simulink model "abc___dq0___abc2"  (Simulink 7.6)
settings: Solver=ode23tb  StartTime=0.0  StopTime=10/f  FixedStep=Ts  RelTol=1e-3
InitFcn:
  | clear all
  | f=60;
  | %Ts=2e-5;
  | clc
  | close all
  | a=exp(j*2*pi/3);
undefined symbols (not defined in the file or in its folder): j
libraries: powerlib_extras x5

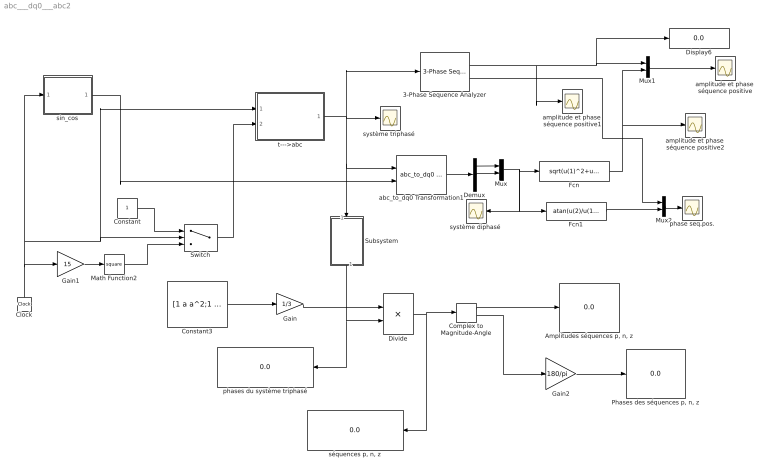
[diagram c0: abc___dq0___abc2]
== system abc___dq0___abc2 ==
  3-Phase Sequence Analyzer : powerlib_extras/Measurements/3-Phase Sequence Analyzer  DialogController=POWERSYS.PowerSysDialog  SystemSampleTime=-1  f1=60  n=1  seq=Positive
  "Amplitudes séquences p, n, z" : Display
  Clock : Clock
  Complex to Magnitude-Angle : ComplexToMagnitudeAngle  SampleTime=0
  Constant : Constant
  Constant3 : Constant  Value=[1 a a^2;1 a^2 a; 1 1 1]
  Demux : Demux  Outputs=3
  Display6 : Display
  Divide : Product  Inputs=**  Multiplication=Matrix(*)
  Fcn : Fcn  Expr=sqrt(u(1)^2+u(2)^2)
  Fcn1 : Fcn  Expr=atan(u(2)/u(1))
  Gain : Gain  Gain=1/3
  Gain1 : Gain  Gain=15
  Gain2 : Gain  Gain=180/pi
  Math Function2 : Math  Operator=square
  Mux : Mux  Inputs=2
  Mux1 : Mux  Inputs=2
  Mux2 : Mux  Inputs=2
  "Phases des séquences p, n, z" : Display
  Subsystem : Subsystem
  Switch : Switch  Threshold=3/f
  abc_to_dq0 Transformation1 : powerlib_extras/Measurements/abc_to_dq0 Transformation  DialogController=POWERSYS.PowerSysDialog  SystemSampleTime=-1
  amplitude et phase  séquence positive : Scope
  amplitude et phase  séquence positive1 : Scope
  amplitude et phase  séquence positive2 : Scope
  phase seq.pos. : Scope
  phases du système triphasé : Display
  sin_cos : Subsystem
  "système diphasé " : Scope
  "système triphasé " : Scope
  "séquences p, n, z" : Display
  t--->abc : Subsystem
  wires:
  t--->abc/1(abc) -> "système triphasé "/1, 3-Phase Sequence Analyzer/1, abc_to_dq0 Transformation1/1, Subsystem/1(syst)
  sin_cos/1(sin_cos) -> abc_to_dq0 Transformation1/2
  Gain1/1 -> Math Function2/1
  Constant/1 -> Switch/1
  Math Function2/1 -> Switch/3
  Switch/1 -> t--->abc/2(a)
  Clock/1 -> Gain1/1, sin_cos/1(t), Switch/2, t--->abc/1(t)
  Fcn1/1 -> Mux2/2
  Mux1/1 -> amplitude et phase  séquence positive/1
  3-Phase Sequence Analyzer/1 -> amplitude et phase  séquence positive1/1, Mux1/1, Display6/1
  Mux2/1 -> phase seq.pos./1
  3-Phase Sequence Analyzer/2 -> Mux2/1
  Fcn/1 -> Mux1/2, amplitude et phase  séquence positive2/1
  abc_to_dq0 Transformation1/1 -> Demux/1
  Demux/1 -> Mux/1
  Mux/1 -> Fcn/1, Fcn1/1, "système diphasé "/1
  Demux/2 -> Mux/2
  Constant3/1 -> Gain/1
  Divide/1 -> Complex to Magnitude-Angle/1, "séquences p, n, z"/1
  Gain/1 -> Divide/1
  Complex to Magnitude-Angle/1 -> "Amplitudes séquences p, n, z"/1
  Complex to Magnitude-Angle/2 -> Gain2/1
  Gain2/1 -> "Phases des séquences p, n, z"/1
  Subsystem/1(cplx) -> Divide/2, phases du système triphasé/1

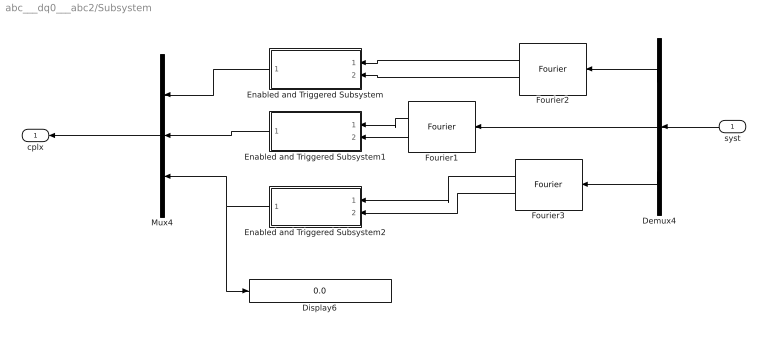
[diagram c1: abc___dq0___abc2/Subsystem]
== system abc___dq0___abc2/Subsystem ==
  syst : Inport
  Demux4 : Demux  Outputs=3
  Display6 : Display
  Enabled and Triggered Subsystem : Subsystem  TreatAsAtomicUnit=on
  Enabled and Triggered Subsystem1 : Subsystem  TreatAsAtomicUnit=on
  Enabled and Triggered Subsystem2 : Subsystem  TreatAsAtomicUnit=on
  Fourier1 : powerlib_extras/Measurements/Fourier  DialogController=POWERSYS.PowerSysDialog  SystemSampleTime=-1  f1=60  n=1
  Fourier2 : powerlib_extras/Measurements/Fourier  DialogController=POWERSYS.PowerSysDialog  SystemSampleTime=-1  f1=60  n=1
  Fourier3 : powerlib_extras/Measurements/Fourier  DialogController=POWERSYS.PowerSysDialog  SystemSampleTime=-1  f1=60  n=1
  Mux4 : Mux  Inputs=3
  cplx : Outport
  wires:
  syst/1 -> Demux4/1
  Demux4/1 -> Fourier2/1
  Demux4/2 -> Fourier1/1
  Demux4/3 -> Fourier3/1
  Fourier2/2 -> Enabled and Triggered Subsystem/2(In2)
  Mux4/1 -> cplx/1
  Fourier2/1 -> Enabled and Triggered Subsystem/1(a1)
  Enabled and Triggered Subsystem/1(a+i b) -> Mux4/1
  Fourier1/1 -> Enabled and Triggered Subsystem1/1(a1)
  Fourier1/2 -> Enabled and Triggered Subsystem1/2(In2)
  Enabled and Triggered Subsystem1/1(a+i b) -> Mux4/2
  Enabled and Triggered Subsystem2/1(a+i b) -> Mux4/3, Display6/1
  Fourier3/1 -> Enabled and Triggered Subsystem2/1(a1)
  Fourier3/2 -> Enabled and Triggered Subsystem2/2(In2)

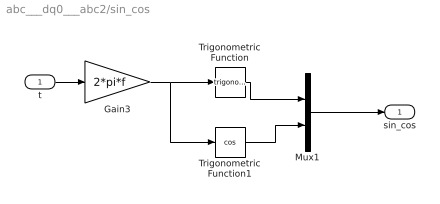
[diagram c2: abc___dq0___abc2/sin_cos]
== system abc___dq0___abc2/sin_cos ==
  t : Inport
  Gain3 : Gain  Gain=2*pi*f
  Mux1 : Mux  Inputs=2
  Trigonometric Function : Trigonometry
  Trigonometric Function1 : Trigonometry  Operator=cos
  sin_cos : Outport
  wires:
  Gain3/1 -> Trigonometric Function/1, Trigonometric Function1/1
  Trigonometric Function/1 -> Mux1/1
  Trigonometric Function1/1 -> Mux1/2
  t/1 -> Gain3/1
  Mux1/1 -> sin_cos/1

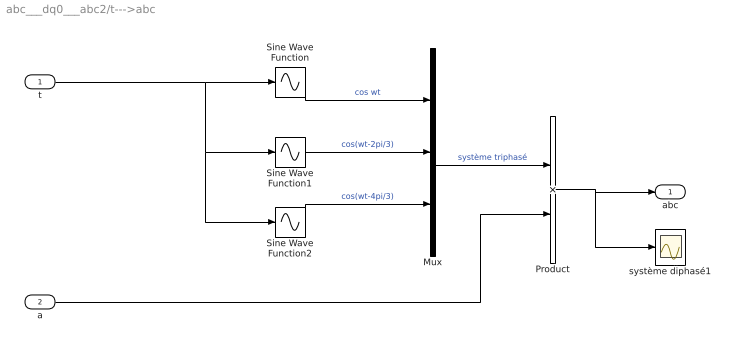
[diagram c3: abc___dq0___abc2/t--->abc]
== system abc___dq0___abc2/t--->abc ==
  t : Inport
  a : Inport  Port=2
  Mux : Mux  Inputs=3
  Product : Product
  Sine Wave Function : Sin  TimeSource=Use external signal  Frequency=2*pi*f  SampleTime=0
  Sine Wave Function1 : Sin  TimeSource=Use external signal  Frequency=2*pi*f  Phase=-2*pi/3  SampleTime=0
  Sine Wave Function2 : Sin  TimeSource=Use external signal  Frequency=2*pi*f  Phase=-4*pi/3  SampleTime=0
  système diphasé1 : Scope
  abc : Outport
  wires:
  Sine Wave Function1/1 -> Mux/2  "cos(wt-2pi/3)"
  Sine Wave Function/1 -> Mux/1  "cos wt"
  Sine Wave Function2/1 -> Mux/3  "cos(wt-4pi/3)"
  t/1 -> Sine Wave Function/1, Sine Wave Function1/1, Sine Wave Function2/1
  Mux/1 -> Product/1  "système triphasé"
  Product/1 -> abc/1, système diphasé1/1
  a/1 -> Product/2

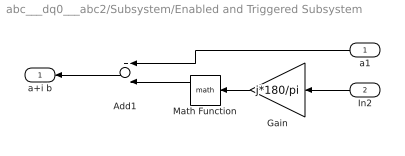
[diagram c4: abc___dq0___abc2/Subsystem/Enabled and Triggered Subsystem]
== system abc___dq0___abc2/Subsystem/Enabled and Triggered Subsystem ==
  a1 : Inport
  In2 : Inport  Port=2
  Add1 : Sum
  Gain : Gain  Gain=j*180/pi
  Math Function : Math
  a+i b : Outport
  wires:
  In2/1 -> Gain/1
  a1/1 -> Add1/1
  Add1/1 -> a+i b/1
  Gain/1 -> Math Function/1
  Math Function/1 -> Add1/2

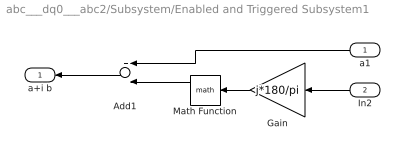
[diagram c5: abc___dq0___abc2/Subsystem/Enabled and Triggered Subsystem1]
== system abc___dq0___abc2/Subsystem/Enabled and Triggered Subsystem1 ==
  a1 : Inport
  In2 : Inport  Port=2
  Add1 : Sum
  Gain : Gain  Gain=j*180/pi
  Math Function : Math
  a+i b : Outport
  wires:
  Math Function/1 -> Add1/2
  Gain/1 -> Math Function/1
  Add1/1 -> a+i b/1
  a1/1 -> Add1/1
  In2/1 -> Gain/1

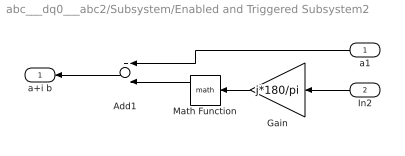
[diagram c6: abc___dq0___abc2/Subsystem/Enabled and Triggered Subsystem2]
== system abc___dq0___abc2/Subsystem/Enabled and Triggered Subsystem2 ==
  a1 : Inport
  In2 : Inport  Port=2
  Add1 : Sum
  Gain : Gain  Gain=j*180/pi
  Math Function : Math
  a+i b : Outport
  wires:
  In2/1 -> Gain/1
  a1/1 -> Add1/1
  Add1/1 -> a+i b/1
  Gain/1 -> Math Function/1
  Math Function/1 -> Add1/2
